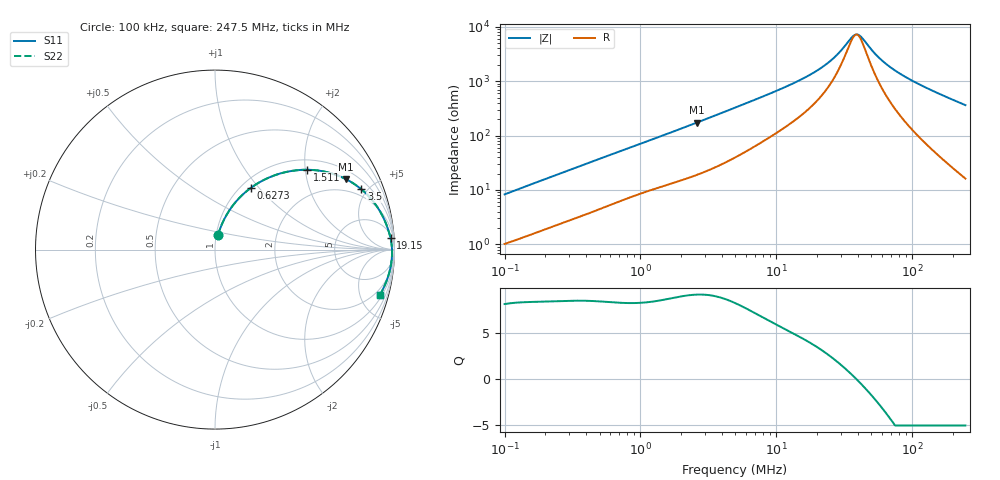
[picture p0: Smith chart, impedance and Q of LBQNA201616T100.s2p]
! LBQNA201616T100  S-PARAMETER MODEL  ( General Type )
! Model Generated by TAIYO YUDEN Corporation (http://www.ty-top.com)
! Version 1.0
! TAIYO YUDEN Control No. 191025NI43SB-FBB
! Copyright(c) 2019 TAIYO YUDEN CO.,LTD. All Rights Reserved.
! Product Description (link to TY-COMPAS)
! https://ds.yuden.co.jp/TYCOMPAS/or/detail?pn=LBQNA201616T100K&u=M
! Products Name : Inductors
! Characteristics :
!  Inductance : 10 uH , SRF(min) : 32 MHz , DC Resistance(max) : 0.65 Ohm
!  Rated Current : Saturation :250 mA , Temp Rise : 270 mA (20 degC)
!  Case Size : 2.0 x 1.6 / 0.079 x 0.063 [mm/inch] , Thickness : 1.6 / 0.063 [mm/inch]
!  (Conditions: Temperature = 25 degC , DC Bias Current/Voltage = 0A / 0V)
! External Node Assignments :
!  1  o---GGG---o  2
! GND o---------o GND
! Frequency Range : 0.1MHz  -  247.502633MHz  [ 402 STEP ]
# MHz S RI R 50
! Freq[MHz].  S11 Real  S11 Imag  S21 Real  S21 Imag  S12 Real  S12 Imag  S22 Real  S22 Imag
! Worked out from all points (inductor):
!   401 points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, 100 kHz to 247.5 MHz, reference 50 ohm
!   read as one part in series: L = 12.9 uH near 104 kHz
!   highest Q = 9.1 at 2.611 MHz (marker M1), where L = 10.5 uH
!   self-resonance near 38.94 MHz
!   S11 on the Smith chart (normalised r, x): 100 kHz: 1.02, +0.16; 627.3 kHz: 1.11, +0.91; 1.511 MHz: 1.24, +2.05; 3.5 MHz: 1.51, +4.57; 19.15 MHz: 9, +28; 247.5 MHz: 1.32, -7.23
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0.1  0.0166 0.08  0.9834 -0.08  0.9834 -0.08  0.0166 0.08
0.194292  0.0399 0.1449  0.9601 -0.1449  0.9601 -0.1449  0.0399 0.1449
0.37019  0.0984 0.2444  0.9016 -0.2444  0.9016 -0.2444  0.0984 0.2444
0.627323  0.2018 0.3454  0.7982 -0.3454  0.7982 -0.3454  0.2018 0.3454
1.370406  0.4737 0.4436  0.5263 -0.4436  0.5263 -0.4436  0.4737 0.4436
1.511016  0.5142 0.4448  0.4858 -0.4448  0.4858 -0.4448  0.5142 0.4448
2.611076  0.7284 0.3932  0.2716 -0.3932  0.2716 -0.3932  0.7284 0.3932
3.500087  0.8155 0.336  0.1845 -0.336  0.1845 -0.336  0.8155 0.336
4.974964  0.8871 0.2613  0.1129 -0.2613  0.1129 -0.2613  0.8871 0.2613
11.08235  0.9601 0.1252  0.0399 -0.1252  0.0399 -0.1252  0.9601 0.1252
18.41681  0.9772 0.0672  0.0228 -0.0672  0.0228 -0.0672  0.9772 0.0672
19.1506  0.978 0.0633  0.022 -0.0633  0.022 -0.0633  0.978 0.0633
26.17735  0.9832 0.0343  0.0168 -0.0343  0.0168 -0.0343  0.9832 0.0343
30.01327  0.9847 0.0223  0.0153 -0.0223  0.0153 -0.0223  0.9847 0.0223
35.78235  0.9859 0.00721  0.0141 -0.00721  0.0141 -0.00721  0.9859 0.00721
38.69052  0.9863 0.000542  0.0137 -0.000542  0.0137 -0.000542  0.9863 0.000542
41.83506  0.9865 -0.00616  0.0135 0.00616  0.0135 0.00616  0.9865 -0.00616
54.99405  0.9863 -0.0303  0.0137 0.0303  0.0137 0.0303  0.9863 -0.0303
68.1772  0.9849 -0.0509  0.0151 0.0509  0.0151 0.0509  0.9849 -0.0509
86.18795  0.9819 -0.0759  0.0181 0.0759  0.0181 0.0759  0.9819 -0.0759
115.5329  0.9749 -0.1126  0.0251 0.1126  0.0251 0.1126  0.9749 -0.1126
247.5026  0.9195 -0.2506  0.0805 0.2506  0.0805 0.2506  0.9195 -0.2506
